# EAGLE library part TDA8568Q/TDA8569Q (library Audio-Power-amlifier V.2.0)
Philips TDA8568Q 4 x 25 W BTL quad car radio power amplifier, TDA8569Q 4 ´ 40 W BTL quad car radio power amplifier http://www.datasheetcatalog.com/datasheets_pdf/T/D/A/8/TDA8568Q.shtml
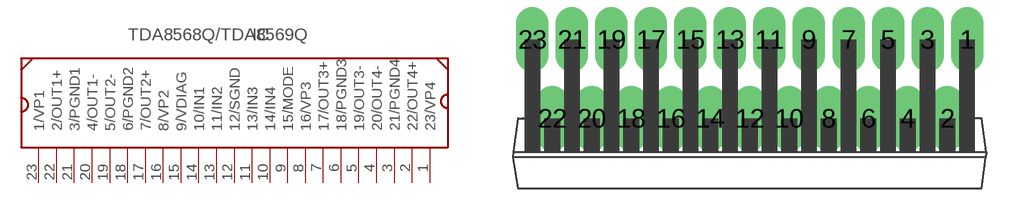
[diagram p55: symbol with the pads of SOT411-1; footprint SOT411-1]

Designator prefix IC

## TDA8568Q/TDA8569Q  [SOT411-1]
1  23/VP4  pwr
2  22/OUT4+  out
3  21/PGND4  pwr
4  20/OUT4-  out
5  19/OUT3-  out
6  18/PGND3  pwr
7  17/OUT3+  out
8  16/VP3  pwr
9  15/MODE
10  14/IN4  in
11  13/IN3  in
12  12/SGND  pwr
13  11/IN2  in
14  10/IN1  in
15  9/VDIAG
16  8/VP2  pwr
17  7/OUT2+  out
18  6/PGND2  pwr
19  5/OUT2-  out
20  4/OUT1-  out
21  3/PGND1  pwr
22  2/OUT1+  out
23  1/VP1  pwr

## Footprint SOT411-1 (pad centres in mm)
drill 1.4 long: 1 13.97,5.08; 2 12.7,0; 3 11.43,5.08; 4 10.16,0; 5 8.89,5.08; 6 7.62,0; 7 6.35,5.08; 8 5.08,0; 9 3.81,5.08; 10 2.54,0; 11 1.27,5.08; 12 0,0; 13 -1.27,5.08; 14 -2.54,0; 15 -3.81,5.08; 16 -5.08,0; 17 -6.35,5.08; 18 -7.62,0; 19 -8.89,5.08; 20 -10.16,0; 21 -11.43,5.08; 22 -12.7,0; 23 -13.97,5.08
